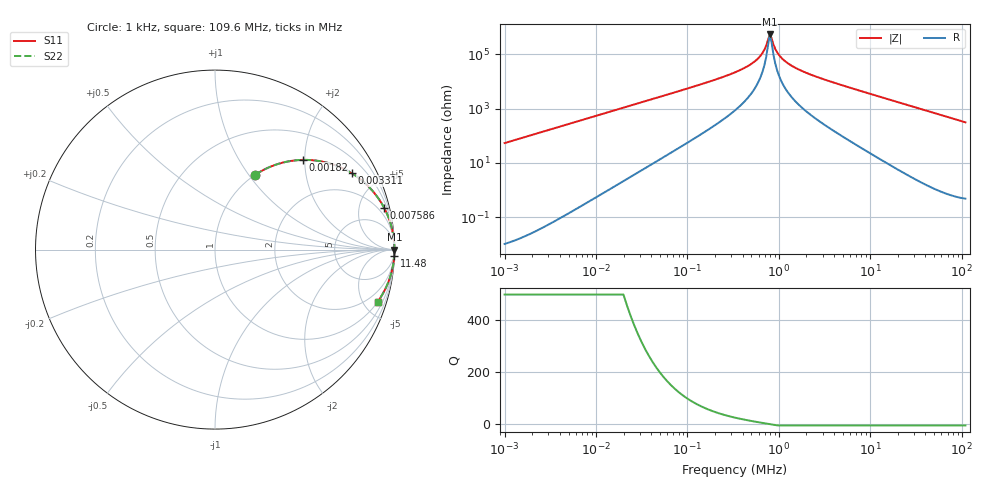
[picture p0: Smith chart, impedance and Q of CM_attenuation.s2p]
! EM Consulting and Software
! Touchstone file was created on 2026-03-09  16:25:52
# HZ S RI R 50.0000
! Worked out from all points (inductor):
!   253 points, 1 kHz to 109.6 MHz, reference 50 ohm
!   read as one part in series: L = 8.57 mH near 1.047 kHz
!   highest |Z| = 531 kohm at 794.3 kHz (marker M1)
!   self-resonance near 794.3 kHz
!   S11 on the Smith chart (normalised r, x): 1 kHz: 1.00, +1.08; 1.82 kHz: 1.00, +1.96; 3.311 kHz: 1.00, +3.57; 7.586 kHz: 1.01, +8.17; 11.48 MHz: 1, -60; 109.6 MHz: 1.01, -6.26
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1000  0.225 0.4175  0.775 -0.4175  0.775 -0.4175  0.225 0.4175
1819.701  0.49 0.4998  0.51 -0.4998  0.51 -0.4998  0.49 0.4998
3311.311  0.7608 0.4264  0.2392 -0.4264  0.2392 -0.4264  0.7608 0.4264
6918.31  0.9327 0.2502  0.0673 -0.2502  0.0673 -0.2502  0.9327 0.2502
7585.776  0.9433 0.2308  0.0567 -0.2308  0.0567 -0.2308  0.9433 0.2308
17378.01  0.9885 0.1055  0.0115 -0.1055  0.0115 -0.1055  0.9885 0.1055
47863.01  0.9983 0.0386  0.00168 -0.0386  0.00168 -0.0386  0.9983 0.0386
331131.1  0.9998 0.00464  0.000207 -0.00464  0.000207 -0.00464  0.9998 0.00464
478630.1  0.9998 0.00249  0.000192 -0.00249  0.000192 -0.00249  0.9998 0.00249
602559.6  0.9998 0.00133  0.000187 -0.00133  0.000187 -0.00133  0.9998 0.00133
691831  0.9998 0.000677  0.000186 -0.000677  0.000186 -0.000677  0.9998 0.000677
724436  0.9998 0.000461  0.000186 -0.000461  0.000186 -0.000461  0.9998 0.000461
794328.2  0.9998 3.34e-05  0.000185 -3.34e-05  0.000185 -3.34e-05  0.9998 3.34e-05
831763.8  0.9998 -0.00018  0.000185 0.00018  0.000185 0.00018  0.9998 -0.00018
912010.8  0.9998 -0.000609  0.000186 0.000609  0.000186 0.000609  0.9998 -0.000609
1096478  0.9998 -0.00149  0.000188 0.00149  0.000188 0.00149  0.9998 -0.00149
1445440  0.9998 -0.00291  0.000194 0.00291  0.000194 0.00291  0.9998 -0.00291
2290868  0.9998 -0.00583  0.000219 0.00583  0.000219 0.00583  0.9998 -0.00583
1.148154e7  0.9987 -0.0331  0.00128 0.0331  0.00128 0.0331  0.9987 -0.0331
1.659587e7  0.9975 -0.0479  0.00249 0.0479  0.00249 0.0479  0.9975 -0.0479
4.786301e7  0.981 -0.1355  0.019 0.1355  0.019 0.1355  0.981 -0.1355
1.096478e8  0.907 -0.2896  0.093 0.2896  0.093 0.2896  0.907 -0.2896
